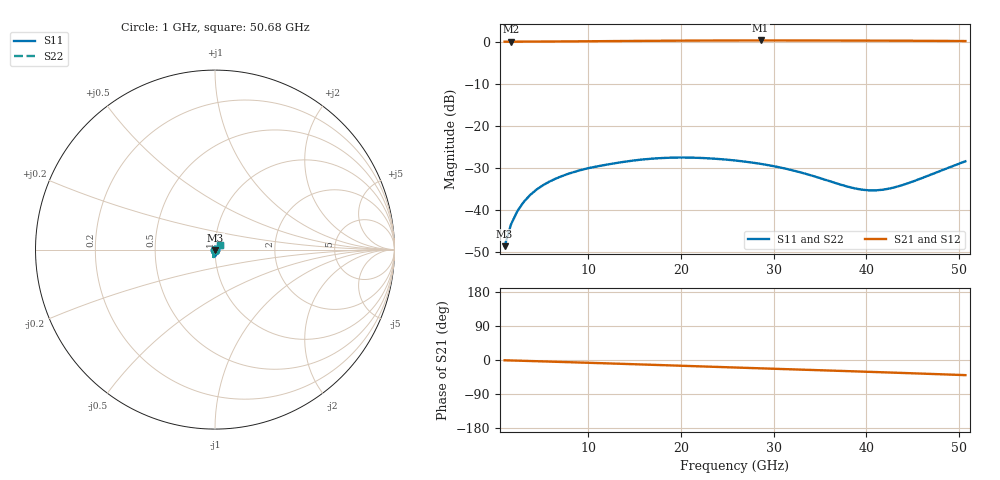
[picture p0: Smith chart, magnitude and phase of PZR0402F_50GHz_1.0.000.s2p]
# GHz S RI R 50
! S-Parameters data
! Freq  reS11  imS11  reS21  imS21  reS12  imS12  reS22  imS22
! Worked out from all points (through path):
!   73 points, 1 GHz to 50.68 GHz, reference 50 ohm
!   highest |S21| = 0.27 dB at 28.6 GHz (marker M1); lowest = 0.0 dB at 1.69 GHz (marker M2)
!   group delay of S21, straight-line fit = 2.19 ps
!   lowest |S11| = -48.7 dB at 1 GHz (marker M3), VSWR 1.01, Z = 50.1 - j0.352 ohm
!   |S11| at or under -10 dB: start of sweep to end of sweep
!   |S22| runs from -48.7 to -27.6 dB; largest |S21 - S12| = 0
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1  0.00107 -0.00352  0.9988 -0.013  0.9988 -0.013  0.00107 -0.00352
1.69  0.00106 -0.00659  0.9985 -0.0214  0.9985 -0.0214  0.00105 -0.00659
2.38  0.000563 -0.0096  0.9986 -0.0296  0.9986 -0.0296  0.000561 -0.0096
3.07  -0.000227 -0.0124  0.9989 -0.0381  0.9989 -0.0381  -0.000223 -0.0124
3.76  -0.00117 -0.0149  0.9993 -0.0468  0.9993 -0.0468  -0.00116 -0.0149
4.45  -0.00218 -0.0172  0.9997 -0.0556  0.9997 -0.0556  -0.00216 -0.0172
5.14  -0.00319 -0.0193  1 -0.0646  1 -0.0646  -0.00317 -0.0193
6.52  -0.00505 -0.0229  1 -0.0826  1 -0.0826  -0.00502 -0.0229
9.28  -0.0078 -0.0287  1.001 -0.1191  1.001 -0.1191  -0.00777 -0.0287
13.42  -0.00958 -0.0352  1 -0.1755  1 -0.1755  -0.00964 -0.0351
17.56  -0.0092 -0.0398  0.9956 -0.2335  0.9956 -0.2335  -0.00931 -0.0397
21.7  -0.00628 -0.0409  0.9858 -0.292  0.9858 -0.292  -0.00647 -0.0408
25.84  -0.00124 -0.0384  0.9701 -0.3493  0.9701 -0.3493  -0.00151 -0.0384
28.6  0.00245 -0.035  0.9566 -0.3863  0.9566 -0.3863  0.00215 -0.035
31.36  0.00591 -0.03  0.9409 -0.4221  0.9409 -0.4221  0.00563 -0.0301
34.81  0.00983 -0.022  0.9186 -0.4654  0.9186 -0.4654  0.0096 -0.0221
37.57  0.0128 -0.0145  0.899 -0.4992  0.899 -0.4992  0.0126 -0.0147
39.64  0.0149 -0.00862  0.8833 -0.5242  0.8833 -0.5242  0.0148 -0.00883
41.02  0.0163 -0.00463  0.8723 -0.5409  0.8723 -0.5409  0.0163 -0.00487
42.4  0.0177 -0.00062  0.8606 -0.5576  0.8606 -0.5576  0.0178 -0.000891
45.16  0.0206 0.00748  0.8353 -0.5902  0.8353 -0.5902  0.0208 0.00714
50.68  0.0284 0.0247  0.7784 -0.6517  0.7784 -0.6517  0.0288 0.0242
